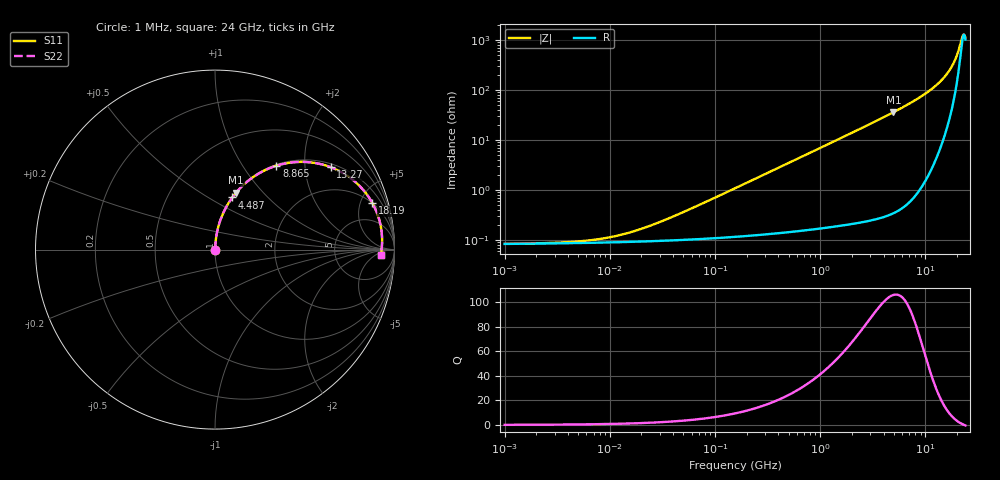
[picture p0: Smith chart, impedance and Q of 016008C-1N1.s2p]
# MHz S MA R 50
!Freq  MagS11  AngS11  MagS21  AngS21  MagS12  AngS12  MagS22  AngS22
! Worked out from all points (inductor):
!   801 points, 1 MHz to 24 GHz, reference 50 ohm
!   read as one part in series: L = 1.1 nH near 42.82 MHz
!   highest Q = 106 at 4.964 GHz (marker M1), where L = 1.15 nH
!   self-resonance near 23.32 GHz
!   S11 on the Smith chart (normalised r, x): 1 MHz: 1.00, +0.00; 4.487 GHz: 1.01, +0.64; 8.865 GHz: 1.02, +1.44; 13.27 GHz: 1.11, +2.72; 18.19 GHz: 2.00, +6.32; 24 GHz: 22, -9
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1  0.00083 4.8  0.9992 -0.0  0.9992 -0.0  0.00083 4.8
2.776492  0.0008671 12.8  0.9992 -0.0  0.9992 -0.0  0.0008671 12.8
5.416084  0.0009414 23.4  0.9991 -0.0  0.9991 -0.0  0.0009414 23.4
8.420146  0.001055 33.4  0.9991 -0.0  0.9991 -0.0  0.001055 33.4
12.60457  0.001251 44.1  0.9991 -0.0  0.9991 -0.0  0.001251 44.1
18.63208  0.001581 54.4  0.9991 -0.1  0.9991 -0.1  0.001581 54.4
28.96647  0.002214 64.5  0.999 -0.1  0.999 -0.1  0.002214 64.5
154.9193  0.01076 83.3  0.9988 -0.6  0.9988 -0.6  0.01076 83.3
839.0561  0.0579 85.1  0.9967 -3.3  0.9967 -3.3  0.0579 85.1
2106.131  0.1449 80.8  0.9874 -8.3  0.9874 -8.3  0.1449 80.8
4487.466  0.3059 71.6  0.9491 -17.8  0.9491 -17.8  0.3059 71.6
4963.674  0.3374 69.7  0.9382 -19.7  0.9382 -19.7  0.3374 69.7
6717.529  0.4503 62.7  0.8883 -26.8  0.8883 -26.8  0.4503 62.7
8864.727  0.5792 53.8  0.807 -35.4  0.807 -35.4  0.5792 53.8
10983.6  0.6918 45.0  0.7068 -43.8  0.7068 -43.8  0.6918 45.0
13270.09  0.7913 35.5  0.5809 -52.3  0.5809 -52.3  0.7913 35.5
15831.7  0.8713 25.2  0.4274 -60.3  0.4274 -60.3  0.8713 25.2
18186.76  0.9146 16.4  0.2858 -64.6  0.2858 -64.6  0.9146 16.4
19864.71  0.9297 10.6  0.1911 -63.2  0.1911 -63.2  0.9297 10.6
22251.52  0.9324 3.1  0.08491 -35.8  0.08491 -35.8  0.9324 3.1
23109.23  0.9292 0.6  0.07149 -7.5  0.07149 -7.5  0.9292 0.6
24000  0.9238 -1.9  0.08242 21.5  0.08242 21.5  0.9238 -1.9
